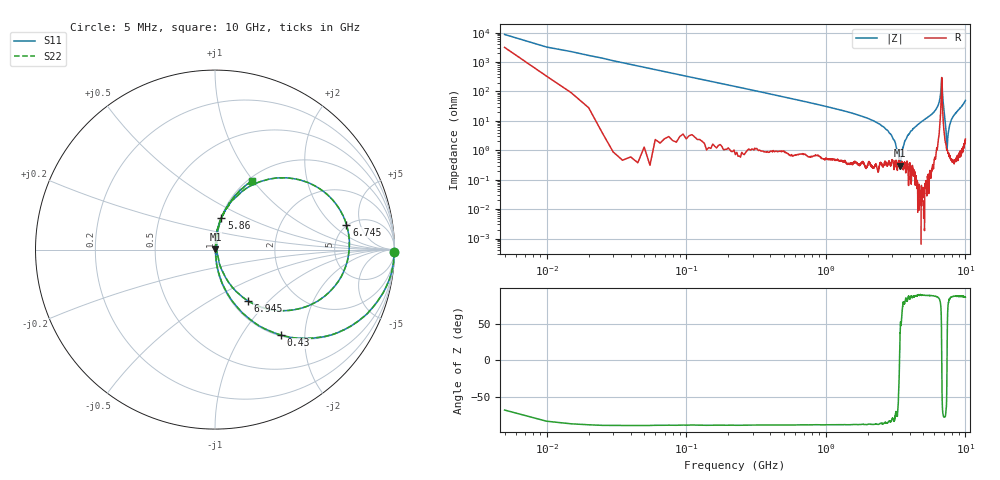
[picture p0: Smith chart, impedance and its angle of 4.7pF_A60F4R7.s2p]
! Amotech Co.,Ltd.
! http://www.amotech.co.kr/
! Part Number: A60F4R7
! These Parameters are Measured in Series Mode Connection
! Operation Temp=25[degC], DC Bias Voltage=0[V]
! Freq. Start=5[MHz] Stop=10[GHz], 2000[Steps]
! Date: Monday, July 20, 2020, 03:26:47
# GHZ S RI R 50.000000
!Freq.(Hz) S11(Real) S11(Imag) S21(Real) S21(Imag) S12(Real) S12(Imag) S22(Real) S22(Imag)
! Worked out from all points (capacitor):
!   2000 points, 5 MHz to 10 GHz, reference 50 ohm
!   read as one part in series: C = 4.84 pF near 55 MHz
!   lowest |Z| = 301 mohm at 3.405 GHz (marker M1)
!   series resonance near 3.376 GHz, so ESL is about 460 pH
!   S11 on the Smith chart (normalised r, x): 5 MHz: open; 430 MHz: 1.02, -1.52; 5.86 GHz: 1.01, +0.37; 6.745 GHz: 4.88, +3.06; 6.945 GHz: 1.18, -0.76; 10 GHz: 1.05, +0.99
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0.005  0.9957 -0.0107  0.0043 0.0107  0.0043 0.0107  0.9957 -0.0107
0.065  0.9618 -0.1901  0.0382 0.1901  0.0382 0.1901  0.9618 -0.1901
0.125  0.8726 -0.329  0.1274 0.329  0.1274 0.329  0.8726 -0.329
0.43  0.3691 -0.4767  0.6309 0.4767  0.6309 0.4767  0.3691 -0.4767
1.675  0.0288 -0.1565  0.9712 0.1565  0.9712 0.1565  0.0288 -0.1565
2.925  0.00438 -0.0345  0.9956 0.0345  0.9956 0.0345  0.00438 -0.0345
3.34  0.00504 -0.00301  0.995 0.00301  0.995 0.00301  0.00504 -0.00301
3.405  0.00237 0.00184  0.9976 -0.00184  0.9976 -0.00184  0.00237 0.00184
3.57  0.00258 0.012  0.9974 -0.012  0.9974 -0.012  0.00258 0.012
3.865  0.00379 0.0315  0.9962 -0.0315  0.9962 -0.0315  0.00379 0.0315
5.005  0.0112 0.1034  0.9888 -0.1034  0.9888 -0.1034  0.0112 0.1034
5.86  0.036 0.1786  0.964 -0.1786  0.964 -0.1786  0.036 0.1786
6.44  0.1461 0.3196  0.8539 -0.3196  0.8539 -0.3196  0.1461 0.3196
6.67  0.5049 0.3781  0.4951 -0.3781  0.4951 -0.3781  0.5049 0.3781
6.745  0.7325 0.1392  0.2675 -0.1392  0.2675 -0.1392  0.7325 0.1392
6.84  0.5223 -0.3121  0.4777 0.3121  0.4777 0.3121  0.5223 -0.3121
6.945  0.1821 -0.2844  0.8179 0.2844  0.8179 0.2844  0.1821 -0.2844
7.21  0.0218 -0.0673  0.9782 0.0673  0.9782 0.0673  0.0218 -0.0673
7.39  0.01 0.000507  0.99 -0.000507  0.99 -0.000507  0.01 0.000507
7.68  0.0111 0.065  0.9889 -0.065  0.9889 -0.065  0.0111 0.065
8.335  0.0296 0.1576  0.9704 -0.1576  0.9704 -0.1576  0.0296 0.1576
10  0.2084 0.3825  0.7916 -0.3825  0.7916 -0.3825  0.2084 0.3825
